FUNCTION_BLOCK FB_Machine
VAR
	// ==============================错误变量=====================================================
	bError				AT%Q*				: BOOL;								// 如果为TRUE，则设备存在错误			（通过输出传递给模拟程序）
	
	// =============================轴相关变量============================================
	fAxisVelo							: LREAL;								// 轴速度，见cAxisVeloAutomatic和cAxisVeloNotAutomatic
		
	// ============================状态机相关变量==================================
	bStarted			AT%Q*				: BOOL;								// 如果为True，则设备进入运行中状态		（通过输出传递给模拟程序）
	bStopped			AT%Q*				: BOOL;								// 如果为True，则设备进入停止状态		（通过输出传递给模拟程序）
	bReset				AT%Q*				: BOOL;								// 如果为True，则设备进入复位中状态		（通过输出传递给模拟程序）
	bAborted			AT%Q*				: BOOL;								// 如果为True，则设备进入中止状态		（通过输出传递给模拟程序）
	bIdle				AT%Q*				: BOOL;								// 如果为True，则设备进入空闲状态		（通过输出传递给模拟程序）
	bAuto				AT%Q*				: BOOL;								// 如果为True，则设备处于自动模式		（通过输出传递给模拟程序）
	bSemi				AT%Q*				: BOOL;								// 如果为True，则设备处于半自动模式		（通过输出传递给模拟程序）
	bManual				AT%Q*				: BOOL;								// 如果为True，则设备处于手动模式		（通过输出传递给模拟程序）
	bMaintenance		AT%Q*				: BOOL;								// 如果为True，则设备处于维护模式		（通过输出传递给模拟程序）
	bStartButtonOff		AT%Q*				: BOOL;								// 如果为True，复位Start按钮			（通过输出传递给模拟程序）

	// =================================对象=======================================
	fbSeparateModule					: FB_SeparatingModule;					// 输送系统
	fbMetalSorting						: FB_SortingModule;						// 金属分拣系统
	fbPlasticSorting					: FB_SortingModule;						// 塑料分拣系统
	fbButtonStart						: FB_SignalHandling;					// 处理启动按钮的信号处理功能块
	fbButtonStop						: FB_SignalHandling;					// 处理停止按钮的信号处理功能块
	fbButtonReset						: FB_SignalHandling;					// 处理复位按钮的信号处理功能块
	fbButtonAbort						: FB_SignalHandling;					// 处理中止按钮的信号处理功能块
	fbButtonAuto						: FB_SignalHandling;					// 处理自动模式按钮的信号处理功能块
	fbButtonSemi						: FB_SignalHandling;					// 处理半自动模式按钮的信号处理功能块
	fbButtonManual						: FB_SignalHandling;					// 处理手动模式按钮的信号处理功能块
	fbButtonMaintenance					: FB_SignalHandling;					// 处理维护模式按钮的信号处理功能块
	fbButtonPower						: FB_SignalHandling;					// 处理使能按钮的信号处理功能块
	fbButtonComprAir					: FB_SignalHandling;					// 处理压缩气缸空气按钮的信号处理功能块
	fbComprAir							: FB_SignalHandling;					// 处理压缩气缸空气的信号处理功能块		（In为fbButtonComprAir的Out）
	fbPowerSupply						: FB_SignalHandling;					// 处理使能的信号处理功能块				（In为fbButtonPower的Out）
	// =================================状态机==========================================
	fbStateMachineAuto					: PS_PackML_StateMachine_Auto;			// 自动模式下的状态机功能块
	fbStateMachineSemiAuto				: PS_PackML_StateMachine_SemiAuto;		// 半自动模式下的状态机功能块
	fbStateMachineManual				: PS_PackML_StateMachine_Manual;		// 手动模式下的状态机功能块
	fbStateMachineMaintenance			: PS_PackML_StateMachine_Maintenance;	// 维护模式下的状态机功能块
	
	ePMLUnitMode						: E_PMLUnitMode := E_PMLUnitMode.IDLE;	// 当前的设备模式
	ePMLUnitModeRequested				: E_PMLUnitMode;						// 请求的设备模式
	fbUnitModeManager					: PS_UnitModeManager;					// 模式切换功能块
	ePMLState							: E_PMLState := E_PMLState.IDLE;		// 当前的设备状态机
	ePMLStateRequested					: E_PMLState;							// 请求的设备状态机
	
	// ===================================其他=====================================
	bInit								: BOOL;									// 如果为TRUE，则设备运行所必须的参数已经初始化完成
	bAxisEnable							: BOOL;									// 如果为TRUE，则轴已经使能
	bManualAxisEnable					: BOOL;									// 如果为TRUE，则轴允许被手动的按钮控制
	fbTriggerStart						: R_TRIG;								// 检测启动按钮的上升沿
	fbTriggerSeparated					: R_TRIG;								// 检测分割完物料的上升沿
	fbTriggerSelectedM					: R_TRIG;								// 检测金属物料被分拣完的上升沿
	fbTriggerSelectedP					: R_TRIG;								// 检测塑料物料被分拣完的上升沿
	nBoxesOnTheWay						: INT;									// 输送带上正在移动的物料
	aClampTemps							: ARRAY[1..100] OF LREAL;				// 正位气缸的温度数据
	aBarrierTemps						: ARRAY[1..100] OF LREAL;				// 栏杆气缸的温度数据
	aMetalTemps							: ARRAY[1..100] OF LREAL;				// 金属气缸的温度数据
	aPlasticTemps						: ARRAY[1..100] OF LREAL;				// 塑料气缸的温度数据
	bStartingIsSetToTrue				: BOOL;									// 如果为TRUE，则启动方法被以TRUE的形式调用
	bResetIsSetToTrue					: BOOL;									// 如果为TRUE，则复位方法被以TRUE的形式调用
	bHaltIsSetToTrue					: BOOL;									// 如果为TRUE，则停止方法被以TRUE的形式调用

	bResetAxis           AT%I*          : BOOL;									// 单独复位轴的报错

END_VAR
VAR CONSTANT
	// ================================轴速度=========================================
	cAxisVeloAutomatic					: LREAL	:= 200.0;						// 自动/半自动模式下轴的运行速度
	cAxisVeloNotAutomatic				: LREAL	:= 100.0;						// 手动/维护模式下轴的运行速度
	
	// ============================= 气缸超时时间参数 =====================================
	cSeparatingTimeOutClamp				: TIME 	:= T#2.5S;						// 正位气缸在位置之间切换判定为超时的时间
	cSeparatingTimeOutBarrier			: TIME 	:= T#3S;						// 栏杆气缸在位置之间切换判定为超时的时间
	cSortingTimeOutCylinder				: TIME 	:= T#3S;						// 分拣气缸在位置之间切换判定为超时的时间
	cSeparatingBarrierAtWork			: TIME 	:= T#3S;						// 栏杆气缸打开的时间
	cSortingMoveAxis					: TIME 	:= T#1S;						// 分拣系统出料皮带运转的时间
	cSortingSensorDelay					: TIME 	:= T#1.4S;						// 对应物料种类传感器检测到之后，到分拣系统气缸推出的延迟时间
END_VAR

// =========================================================
// 关联报错
	
	bError := fbSeparateModule.bAxisError OR fbSeparateModule.bClampError OR fbSeparateModule.bBarrierError
			OR fbMetalSorting.bAxisError OR fbMetalSorting.bCylError 
			OR fbPlasticSorting.bAxisError OR fbPlasticSorting.bCylError;
	
// =========================================================
// 根据不同的模式选择对应轴的速度

	IF (ePMLUnitMode = E_PMLUnitMode.AUTOMATIC) OR (ePMLUnitMode = E_PMLUnitMode.SEMIAUTOMATIC) THEN
		fAxisVelo := cAxisVeloAutomatic;
	ELSE
		fAxisVelo := cAxisVeloNotAutomatic;
	END_IF

// =========================================================
// 检测子系统当中的标志位信号
	
	fbTriggerSeparated(CLK := fbSeparateModule.bSeparated);			// 分割物料完成
	fbTriggerSelectedM(CLK := fbMetalSorting.bSelected);			// 金属物料分拣完成
	fbTriggerSelectedP(CLK := fbPlasticSorting.bSelected);			// 塑料物料分拣完成
						
// =========================================================
// 关联温度
	
	aBarrierTemps 	:= fbSeparateModule.aBarrierTemps;				
	aClampTemps 	:= fbSeparateModule.aClampTemps;
	aMetalTemps 	:= fbMetalSorting.aTemps;
	aPlasticTemps 	:= fbPlasticSorting.aTemps;

// =========================================================
// 方法调用

	// 初始化
	General_Init();

	// 设备请求
	General_Requests();
	
	// 使能、气缸压缩、信号处理功能块的启用
	General_Enable();
	
	// 关联输入
	General_ModuleInputs();
	
	// 关联输出
	General_SetOutput();
	
	// 状态机处理
	General_StateMachine();
	
	// 内部检查
	CylicCheckInternal();
	
	// 复位轴报错（MC_Reset）
	fbSeparateModule.R_Axis.Reset(bResetAxis);
    fbMetalSorting  .R_Axis.Reset(bResetAxis);
	fbPlasticSorting.R_Axis.Reset(bResetAxis);

METHOD PRIVATE CylicCheckInternal
VAR_INPUT
END_VAR


fbSeparateModule.CylicCheck();		// 输送系统内部检查


fbMetalSorting.CylicCheck();		// 金属分拣系统内部检查


fbPlasticSorting.CylicCheck();		// 塑料分拣系统内部检查
END_METHOD

METHOD PRIVATE General_Enable
VAR_INPUT
END_VAR
// =========================================================
// 使能处理

	fbButtonPower.Enable(bEnable := TRUE);			// 启用使能按钮
	fbPowerSupply.Enable(bEnable := TRUE);			// 启用使能按钮输出的信号
	
	fbPowerSupply.bInput := fbButtonPower.bOut;		// 将使能按钮信号的输出传递给使能信号功能块的输入

// =========================================================
// 轴控使能、手动的标志位处理
	
	// 如果设备进入中止状态，则轴使能自动解除							
	IF (ePMLState = E_PMLState.ABORTED) THEN
		bAxisEnable := FALSE;
		
	// 如果使能信号功能块的输出为TRUE，则bAxisEnable为TRUE
	ELSIF fbPowerSupply.bOut THEN
		bAxisEnable := TRUE;
	END_IF
	
	// 允许轴的手动控制：条件：使能上且设备处于运行状态和手动/自动模式
	bManualAxisEnable := fbPowerSupply.bOut AND (ePMLState = E_PMLState.EXECUTE)
						AND ((ePMLUnitMode = E_PMLUnitMode.MANUAL) OR (ePMLUnitMode = E_PMLUnitMode.MAINTENANCE));
						
// =========================================================
// 气缸压缩处理
	
	// 如果不是维护模式，那使能信号的输出传递给气缸加压信号功能块的输入（随着使能信号的输出自动加压）
	IF (ePMLUnitMode <> E_PMLUnitMode.MAINTENANCE) THEN
		fbComprAir.bInput := fbPowerSupply.bOut;
		
	//	气缸加压按钮信号功能块的输出传递给气缸加压信号功能块的输入
	ELSE
		fbComprAir.bInput := fbButtonComprAir.bOut;
	END_IF
	
	// 保持气缸加压信号功能块启用
	fbComprAir.Enable(bEnable := TRUE);
	
	// 维护模式下启用气缸加压按钮信号功能块
	fbButtonComprAir.Enable(bEnable := (ePMLUnitMode = E_PMLUnitMode.MAINTENANCE));

// =========================================================
// 输送系统使能方法的调用

	fbSeparateModule.Enable(bComprAirEnabled	:= fbComprAir.bOut,
							bAxisEnable			:= bAxisEnable,
							bSensorEnable		:= TRUE,
							bManualAxisEnable	:= bManualAxisEnable);

// =========================================================
// 金属分拣系统使能方法的调用

	fbMetalSorting.Enable(	bComprAirEnabled	:= fbComprAir.bOut,
							bAxisEnable			:= bAxisEnable,
							bSensorEnable		:= TRUE,
							bManualAxisEnable	:= bManualAxisEnable);

// =========================================================
// 塑料分拣系统使能方法的调用

	fbPlasticSorting.Enable(bComprAirEnabled	:= fbComprAir.bOut,
							bAxisEnable			:= bAxisEnable,
							bSensorEnable		:= TRUE,
							bManualAxisEnable	:= bManualAxisEnable);

// =========================================================
// 其他信号处理功能块的启用
		
	// 启动按钮：（设备非空闲状态且设备无错误）
	fbButtonStart.Enable(bEnable		:= NOT ((ePMLState = E_PMLState.IDLE) AND bError));
	
	// 停止按钮：（设备运行以及空闲状态下都可以进行停止）
	fbButtonStop.Enable(bEnable 		:= (ePMLState = E_PMLState.EXECUTE) OR (ePMLState = E_PMLState.IDLE));
	
	// 复位按钮：（设备在停止状态下才会被启用）
	fbButtonReset.Enable(bEnable		:= (ePMLState = E_PMLState.STOPPED));
	
	// 使能信号功能块的输出取反传递给中止信号功能块的输入（中止即代表设备掉使能）
	fbButtonAbort.bInput 				:= NOT fbPowerSupply.bOut;
	
	// 中止按钮：（设备在执行、停止中或者复位中才会被启用）
	fbButtonAbort.Enable(bEnable 		:= (ePMLState = E_PMLState.EXECUTE) OR (ePMLState = E_PMLState.STOPPING) OR (ePMLState = E_PMLState.RESETTING));
								
	// 自动模式按钮：（设备在空闲状态下且当前模式非自动模式）
	fbButtonAuto.Enable(bEnable 		:= (ePMLState = E_PMLState.IDLE) AND (ePMLUnitMode <> E_PMLUnitMode.AUTOMATIC));
	
	// 半自动模式按钮：（设备在空闲状态下且当前模式非半自动模式）
	fbButtonSemi.Enable(bEnable 		:= (ePMLState = E_PMLState.IDLE) AND (ePMLUnitMode <> E_PMLUnitMode.SEMIAUTOMATIC));
	
	// 手动模式按钮：（设备在空闲状态下且当前模式非手动模式）
	fbButtonManual.Enable(bEnable 		:= (ePMLState = E_PMLState.IDLE) AND (ePMLUnitMode <> E_PMLUnitMode.MANUAL));
	
	// 维护模式按钮：（设备在空闲状态下且当前模式非维护模式）
	fbButtonMaintenance.Enable(bEnable	:= (ePMLState = E_PMLState.IDLE) AND (ePMLUnitMode <> E_PMLUnitMode.MAINTENANCE));

// =========================================================
END_METHOD

METHOD PRIVATE General_Init
VAR_INPUT
END_VAR
// =========================================================

IF NOT bInit THEN
	
	// 各个子系统的执行必要参数，这些参数都是固定参数，所以只需要传递一次即可
		
		// 传递输送系统正位气缸的超时时间
		fbSeparateModule.tTimeOutOfClamp 			:= cSeparatingTimeOutClamp;
		
		// 传递输送系统栏杆气缸的超时时间
		fbSeparateModule.tTimeOutOfBarrier 			:= cSeparatingTimeOutBarrier;
		
		// 传递输送系统栏杆气缸维持在目标位（打开）的时间
		fbSeparateModule.tBarrierAtWorkPos			:= cSeparatingBarrierAtWork;

		// 传递金属分拣系统正位气缸的超时时间
		fbMetalSorting.tTimeOutOfCylinder 			:= cSortingTimeOutCylinder;		
		
		// 传递金属分拣系统出料皮带运转的时间
		fbMetalSorting.tAxisMovement 				:= cSortingMoveAxis;
		
		// 传递金属物料传感器检测到之后，到金属分拣系统气缸推出的延迟时间
		fbMetalSorting.tDelayOfSensor 				:= cSortingSensorDelay;
		
		// 传递塑料分拣系统正位气缸的超时时间
		fbPlasticSorting.tTimeOutOfCylinder 		:= cSortingTimeOutCylinder;
		
		// 传递塑料分拣系统出料皮带运转的时间
		fbPlasticSorting.tAxisMovement 				:= cSortingMoveAxis;
		
		// 传递塑料物料传感器检测到之后，到塑料分拣系统气缸推出的延迟时间
		fbPlasticSorting.tDelayOfSensor 			:= cSortingSensorDelay;

	// 初始化只执行一次
		bInit := TRUE;
END_IF

// =========================================================
END_METHOD

METHOD PRIVATE General_ModuleInputs
VAR_INPUT
END_VAR
// =========================================================
// 输送系统

	// 如果设备状态为运行状态，则输送系统的bExecute被置为TRUE
	fbSeparateModule.bExecute 			:= (ePMLState = E_PMLState.EXECUTE);
	
	// 每按下一次bStart按钮，输送系统的bSemiStart被置为TRUE，从而保证在半自动模式下，每按下一次bStart启动一次分拣周期
	fbSeparateModule.bSemiStart 		:= fbTriggerStart.Q;
	
	// 传递设定速度到输送系统（运输皮带）当中
	fbSeparateModule.fAxisVelocity 	:= fAxisVelo;

	// 传递皮带上物料的数量到输送系统当中
	fbSeparateModule.nBoxesOnTheWay 	:= nBoxesOnTheWay;
	
	// 通过两个分拣系统物料检测传感器延迟的输出从而判断物料已经到达对应的推出气缸正下方（用于暂停输送皮带的运转）
	fbSeparateModule.P_BoxUndertheCylinderPosition	:= fbPlasticSorting.fbSensorDelay.bOut 		 OR fbMetalSorting .fbSensorDelay.bOut;
	
	// 通过两个分拣系统推出气缸的到达目标位置标志位从而判断对应物料的推出气缸已经工作完成（用于重新启用输送皮带）
	fbSeparateModule.P_CylinderWorkDone				:= fbPlasticSorting.bState_CylinderAtWorkPos OR fbMetalSorting.bState_CylinderAtWorkPos;

// =========================================================
// 金属分拣系统
	
	// 传递设定速度到金属分拣系统（金属出料皮带）当中
	fbMetalSorting.fAxisVelocity 	:= fAxisVelo;

// =========================================================
// 塑料分拣系统

	// 传递设定速度到塑料分拣系统（塑料出料皮带）当中
	fbPlasticSorting.fAxisVelocity 	:= fAxisVelo;
	
// =========================================================
END_METHOD

METHOD PRIVATE General_Requests
VAR_INPUT
END_VAR
// ============================模式=============================

	// 检测启动按钮上升沿
	fbTriggerStart( CLK := fbButtonStart.bOut);
	
	// 如果关闭启动按钮为TRUE，且外部没用按下启动按钮，那么关闭启动按钮自动回归FALSE
	IF bStartButtonOff AND NOT fbButtonStart.bInput THEN
		bStartButtonOff := FALSE;
	END_IF
	
	// 如果检测到启动按钮的上升沿，那么将关闭启动按钮置为TRUE，也只有启动置回，才能将对应的状态传递给ePMLStateRequested
	IF fbTriggerStart.Q THEN
		bStartButtonOff := TRUE;
		
		// 如果设备被中止了，那么状态的请求则为需要清除中
		IF ePMLState = E_PMLState.ABORTED THEN
			ePMLStateRequested := E_PMLState.CLEARING;
		
		// 如果设备停止了，那么状态的请求则为需要复位中	
		ELSIF ePMLState = E_PMLState.STOPPED THEN
			ePMLStateRequested := E_PMLState.RESETTING;
		
		// 如果设备的状态为空闲，且设备已经使能上，那么状态的请求则为需要启动中	
		ELSIF ePMLState = E_PMLState.IDLE AND fbPowerSupply.bOut THEN
			ePMLStateRequested := E_PMLState.STARTING;
		END_IF
		
	// 即使设备没有接收到启动的指令，如果停止按钮按下，那么状态的请求则为需要停止中	
	ELSIF fbButtonStop.bOut THEN
		ePMLStateRequested := E_PMLState.STOPPING;
	
	// 	即使设备没有接收到启动的指令，如果复位按钮按下，那么状态的请求则为需要复位中	
	ELSIF fbButtonReset.bOut THEN
		ePMLStateRequested := E_PMLState.RESETTING;
	END_IF

// ============================状态=============================

	// 如果手动模式按钮按下，那么模式的请求则为手动模式	
	IF fbButtonManual.bOut THEN
		ePMLUnitModeRequested := E_PMLUnitMode.MANUAL;
	
	// 如果自动模式按钮按下，那么模式的请求则为自动模式		
	ELSIF fbButtonAuto.bOut THEN
		ePMLUnitModeRequested := E_PMLUnitMode.AUTOMATIC;
	
	// 如果半自动模式按钮按下，那么模式的请求则为半自动模式		
	ELSIF fbButtonSemi.bOut THEN
		ePMLUnitModeRequested := E_PMLUnitMode.SEMIAUTOMATIC;
	
	// 如果维护模式按钮按下，那么模式的请求则为维护模式		
	ELSIF fbButtonMaintenance.bOut THEN
		ePMLUnitModeRequested := E_PMLUnitMode.MAINTENANCE;
	END_IF
	
	// 如果有任何一个模式按钮的输出模拟，那么会调用模式切换功能块进行模式的切换
	IF fbButtonManual.bOut OR fbButtonAuto.bOut OR fbButtonSemi.bOut OR fbButtonMaintenance.bOut THEN
		fbUnitModeManager(	Execute 		:= TRUE,
							eModeCommand 	:= ePMLUnitModeRequested,
							ePMLState 		:= ePMLState);
	END_IF
	
	// 完成模式切换之后，从模式切换功能块当中传递输出到本地，并将模式切换功能块的Execute置回FALSE
	IF fbUnitModeManager.Done THEN
		ePMLUnitMode := fbUnitModeManager.eModeStatus;
		
		fbUnitModeManager(Execute := FALSE);
	END_IF
	
// =========================================================
END_METHOD

METHOD PRIVATE General_SetOutput
VAR_INPUT
END_VAR
// =========================================================
// 根据PackML状态的枚举体值输出对应的状态标志位

	bStopped 		:= (ePMLState = E_PMLState.STOPPED);
	bStarted 		:= (ePMLState = E_PMLState.EXECUTE);
	bReset 			:= (ePMLState = E_PMLState.RESETTING);
	bAborted 		:= (ePMLState = E_PMLState.ABORTED);
	bIdle 			:= (ePMLState = E_PMLState.IDLE AND fbPowerSupply.bOut);

// =========================================================
// 根据PackML模式的枚举体值输出对应的模式标志位

	bAuto 			:= (ePMLUnitMode = E_PMLUnitMode.AUTOMATIC);
	bSemi 			:= (ePMLUnitMode = E_PMLUnitMode.SEMIAUTOMATIC);
	bManual 		:= (ePMLUnitMode = E_PMLUnitMode.MANUAL);
	bMaintenance 	:= (ePMLUnitMode = E_PMLUnitMode.MAINTENANCE);

// =========================================================
// 输出使能以及压缩气缸信号处理功能块
		
	fbPowerSupply.SetOutput();
	fbComprAir.SetOutput();		

// =========================================================
// 调用各个子系统的输入输出关联方法

	fbSeparateModule.InputOutput();
	fbMetalSorting.InputOutput();
	fbPlasticSorting.InputOutput();

// =========================================================
// 输出各个按钮信号功能块

	fbButtonPower.SetOutput();
	fbButtonComprAir.SetOutput();	
	fbButtonStart.SetOutput();
	fbButtonStop.SetOutput();
	fbButtonReset.SetOutput();
	fbButtonAbort.SetOutput();
	fbButtonAuto.SetOutput();
	fbButtonSemi.SetOutput();
	fbButtonManual.SetOutput();
	fbButtonMaintenance.SetOutput();	
	
// =========================================================
END_METHOD

METHOD PRIVATE General_StateMachine
VAR_INPUT
END_VAR
// =========================================================
	// 模式处理
	
CASE ePMLUnitMode OF
	
	// =========================================================	
	E_PMLUnitMode.AUTOMATIC:		
										  // ePMLStateRequested为 STARTING（在按下启动按钮的时）
				fbStateMachineAuto(	      Start 	:= ePMLStateRequested = E_PMLState.STARTING,	
					
										  // 按下停止按钮时						
									      Stop 	    := fbButtonStop.bOut,	
									
										  // 按下复位按钮时，或者ePMLStateRequested为 RESETTING（停止状态下再次按下启动也可触发）			
									      Reset 	:= fbButtonReset.bOut OR ePMLStateRequested = E_PMLState.RESETTING,		
										  
										  // ePMLStateRequested为 CLEARING（中止状态下按下启动按钮时）
									      Clear 	:= ePMLStateRequested = E_PMLState.CLEARING,				

										  // 按下中止按钮时，或设备在运行的时候出现错误			
									      Abort   	:= fbButtonAbort.bOut OR (bError AND ePMLState = E_PMLState.EXECUTE),	
										  
                                          ePMLState => ePMLState );

				
				Operating_Automatic();

	// =========================================================	
	E_PMLUnitMode.MANUAL:	
	
				// 同上
				fbStateMachineManual(     Start 	:= ePMLStateRequested = E_PMLState.STARTING,
										  Stop 	    := fbButtonStop.bOut,
										  Reset 	:= fbButtonReset.bOut OR ePMLStateRequested = E_PMLState.RESETTING,
										  Clear 	:= ePMLStateRequested = E_PMLState.CLEARING,
										  Abort 	:= fbButtonAbort.bOut OR (bError AND ePMLState = E_PMLState.EXECUTE),
                                          ePMLState => ePMLState);

				
				Operating_Manual();
	
	// =========================================================						
	E_PMLUnitMode.SEMIAUTOMATIC:	

				// 同上
				fbStateMachineSemiAuto(	  Start 	:= ePMLStateRequested = E_PMLState.STARTING,
									 	  Stop 	    := fbButtonStop.bOut,
										  Reset 	:= fbButtonReset.bOut OR ePMLStateRequested = E_PMLState.RESETTING,
										  Clear 	:= ePMLStateRequested = E_PMLState.CLEARING,
										  Abort 	:= fbButtonAbort.bOut OR (bError AND ePMLState = E_PMLState.EXECUTE),
                                          ePMLState => ePMLState);

				
				Operating_Semiautomatic();
	
	// =========================================================						
	E_PMLUnitMode.MAINTENANCE:	

				// 同上
				fbStateMachineMaintenance(Start 	:= ePMLStateRequested = E_PMLState.STARTING,
										  Stop      := fbButtonStop.bOut,
										  Reset 	:= fbButtonReset.bOut OR ePMLStateRequested = E_PMLState.RESETTING,
										  Clear 	:= ePMLStateRequested = E_PMLState.CLEARING,
										  Abort 	:= fbButtonAbort.bOut OR (bError AND ePMLState = E_PMLState.EXECUTE),
                                          ePMLState => ePMLState);

				
				Operating_Maintenance();
END_CASE

// =========================================================
END_METHOD

METHOD PRIVATE Operating_Automatic
VAR_INPUT
END_VAR
// =========================================================

CASE ePMLState OF
	
	// ========================空闲状态=================================
	E_PMLState.IDLE:
	
				// 如果上一个周期中，是用复位来进入空闲状态时，那么先让各个子系统的复位方法以FALSE的形式调用。顺便将StateComplete置回FALSE
				IF bResetIsSetToTrue THEN
					bResetIsSetToTrue := FALSE;
					
					fbSeparateModule.Reset(bReset := FALSE);							
					fbMetalSorting.Reset(bReset := FALSE);
					fbPlasticSorting.Reset(bReset := FALSE);
					
					fbStateMachineAuto.StateComplete := FALSE;	
				END_IF
	
	// ========================启动中状态================================
	E_PMLState.STARTING:
	
				// 以TRUE的形式调用各个子系统的Starting方法
				IF NOT bStartingIsSetToTrue THEN
					bStartingIsSetToTrue := TRUE;
					
					fbSeparateModule.Starting(bStarting := TRUE);
					fbMetalSorting.Starting(bStarting := TRUE);
					fbPlasticSorting.Starting(bStarting := TRUE);
				END_IF
				
				// 如果各个子系统未完成启动的流程，则继续以TRUE的形式调用各个子系统的Starting方法
				IF NOT fbSeparateModule.bState_StartingDone THEN		
					fbSeparateModule.Starting(bStarting := TRUE);
				END_IF	
				IF NOT fbMetalSorting.bState_StartingDone THEN
					fbMetalSorting.Starting(bStarting := TRUE);
				END_IF				
				IF NOT fbPlasticSorting.bState_StartingDone THEN
					fbPlasticSorting.Starting(bStarting := TRUE);
				END_IF

				// 如果所有子系统都完成了启动，那StateComplete则为TRUE。代表启动完成。状态会经过状态机功能块自动进入EXECUTE
				IF fbSeparateModule.bState_StartingDone AND fbMetalSorting.bState_StartingDone AND fbPlasticSorting.bState_StartingDone THEN
					fbStateMachineAuto.StateComplete := TRUE;
				END_IF

	// ==========================执行中状态===============================
	E_PMLState.EXECUTE:	
				
				// 进入运行状态之后，先将bStartingIsSetToTrue置为FALSE，再将各个子系统的启动方法以FALSE调用，同时StateComplete置为FALSE
				IF bStartingIsSetToTrue THEN
					bStartingIsSetToTrue := FALSE;
					
					fbSeparateModule.Starting(bStarting := FALSE);
					fbMetalSorting.Starting(bStarting := FALSE);	
					fbPlasticSorting.Starting(bStarting := FALSE);
					
					fbStateMachineAuto.StateComplete := FALSE;
				END_IF
				
				// 调用各个子系统的自动方法
				fbSeparateModule.Automatic();
				fbMetalSorting.Automatic();
				fbPlasticSorting.Automatic();
				
				// 如果检测到被分割物料的上升沿，那么nBoxesOnTheWay会加1，代表输送带上有一个物料正在运输
				IF fbTriggerSeparated.Q THEN
					nBoxesOnTheWay := nBoxesOnTheWay + 1;
				END_IF
				
				// 如果检测到金属物料被分拣完成的上升沿，那么nBoxesOnTheWay会减1，代表输送带上少了一个正在运输的物料
				IF fbTriggerSelectedM.Q THEN
					nBoxesOnTheWay := nBoxesOnTheWay - 1;
				END_IF
				
				// 如果检测到塑料物料被分拣完成的上升沿，那么nBoxesOnTheWay会减1，代表输送带上少了一个正在运输的物料
				IF fbTriggerSelectedP.Q THEN
					nBoxesOnTheWay := nBoxesOnTheWay - 1;
				END_IF
						
	// =========================中止中状态================================
	E_PMLState.ABORTING:

				// 进入中止中状态之后，先将bHaltIsSetToTrue置为TRUE，再将各个子系统的Halt方法以TRUE调用
				IF NOT bHaltIsSetToTrue THEN
					bHaltIsSetToTrue := TRUE;
					
					fbSeparateModule.Halt(bHalt := TRUE);
					fbMetalSorting.Halt(bHalt := TRUE);
					fbPlasticSorting.Halt(bHalt := TRUE);
				END_IF

				// 如果各个子系统未完成停止的流程，则继续以TRUE的形式继续调用各个子系统的Halt方法
				IF NOT fbSeparateModule.bState_HaltDone THEN
					fbSeparateModule.Halt(bHalt := TRUE);
				END_IF		
				IF NOT fbMetalSorting.bState_HaltDone THEN
					fbMetalSorting.Halt(bHalt := TRUE);
				END_IF				
				IF NOT fbPlasticSorting.bState_HaltDone THEN
					fbPlasticSorting.Halt(bHalt := TRUE);
				END_IF

				// 如果所有子系统都停止了，那StateComplete则为TRUE。代表中止完成。状态会经过状态机功能块自动进入ABORTED
				IF fbSeparateModule.bState_HaltDone AND fbMetalSorting.bState_HaltDone AND fbPlasticSorting.bState_HaltDone THEN
					fbStateMachineAuto.StateComplete := TRUE;
				END_IF
	
	// ========================中止状态=================================
	E_PMLState.ABORTED:
				
				// 进入中止状态之后，先将bHaltIsSetToTrue置回FALSE，再将各个子系统的Halt方法以FALSE调用
				IF bHaltIsSetToTrue THEN
					bHaltIsSetToTrue := FALSE;
					
					fbSeparateModule.Halt(bHalt := FALSE);
					fbMetalSorting.Halt(bHalt := FALSE);
					fbPlasticSorting.Halt(bHalt := FALSE);
				END_IF
				
				// 将StateComplete置回FALSE
				IF fbStateMachineAuto.StateComplete THEN
					fbStateMachineAuto.StateComplete := FALSE;
				END_IF
	
	// =======================清除中状态================================
	E_PMLState.CLEARING:
				
				// 将StateComplete置为TRUE，这里清除中的过程是用Reseting代替
				fbStateMachineAuto.StateComplete := TRUE;
	
	// =========================正常的停止中状态================================
	E_PMLState.STOPPING:	
				
				// 如果检测到被分割物料的上升沿，那么nBoxesOnTheWay会加1，代表输送带上有一个物料正在运输
				IF fbTriggerSeparated.Q THEN
					nBoxesOnTheWay := nBoxesOnTheWay + 1;
				END_IF		
		
				// 如果检测到金属物料被分拣完成的上升沿，那么nBoxesOnTheWay会减1，代表输送带上少了一个正在运输的物料
				IF fbTriggerSelectedM.Q THEN
					nBoxesOnTheWay := nBoxesOnTheWay - 1;
				END_IF
				
				// 如果检测到塑料物料被分拣完成的上升沿，那么nBoxesOnTheWay会减1，代表输送带上少了一个正在运输的物料
				IF fbTriggerSelectedP.Q THEN
					nBoxesOnTheWay := nBoxesOnTheWay - 1;
				END_IF
				
					// 只有当nBoxesOnTheWay为0且bHaltIsSetToTrue为FALSE（没用以TRUE调用过Halt方法）的时候，将bHaltIsSetToTrue置为TRUE
				IF (nBoxesOnTheWay = 0) AND NOT bHaltIsSetToTrue THEN
					bHaltIsSetToTrue := TRUE;
				END_IF
				
				// 如果输送系统没用完成停止，或者输送带上仍然有物料，那么继续调用输送系统的自动方法等待该流程执行完毕。当nBoxesOnTheWay为0，以TRUE调用输送系统的Halt方法
				IF NOT fbSeparateModule.bState_HaltDone OR (nBoxesOnTheWay <> 0) THEN
					fbSeparateModule.Automatic();
					
					IF (nBoxesOnTheWay = 0) THEN
						fbSeparateModule.Halt(bHalt := TRUE);
					END_IF
				END_IF
				
				// 如果输送系统没用完成停止，或者输送带上仍然有物料，那么继续调用输送系统的自动方法等待该流程执行完毕。当nBoxesOnTheWay为0，以TRUE调用金属分拣系统的Halt方法
				IF NOT fbMetalSorting.bState_HaltDone OR (nBoxesOnTheWay <> 0) THEN
					fbMetalSorting.Automatic();
					
					IF (nBoxesOnTheWay = 0) THEN
						fbMetalSorting.Halt(bHalt := TRUE);
					END_IF
				END_IF
				
				// 如果输送系统没用完成停止，或者输送带上仍然有物料，那么继续调用输送系统的自动方法等待该流程执行完毕。当nBoxesOnTheWay为0，以TRUE调用塑料分拣系统的Halt方法
				IF NOT fbPlasticSorting.bState_HaltDone OR (nBoxesOnTheWay <> 0) THEN
					fbPlasticSorting.Automatic();
					
					IF (nBoxesOnTheWay = 0) THEN
						fbPlasticSorting.Halt(bHalt := TRUE);
					END_IF
				END_IF
				
				// 如果各个子系统都完成停止了，且输送带上没有物料了，StateComplete才会被置为TRUE，代表停止完成。状态会经过状态机功能块自动进入STOPPED
				IF fbSeparateModule.bState_HaltDone AND fbMetalSorting.bState_HaltDone
				AND fbPlasticSorting.bState_HaltDone AND (nBoxesOnTheWay = 0) THEN
					fbStateMachineAuto.StateComplete := TRUE;
				END_IF
					
	// ===========================停止状态==============================
	E_PMLState.STOPPED:	

				// 进入停止状态之后，先将bHaltIsSetToTrue置回FALSE，再将各个子系统的Halt方法以FALSE调用
				IF bHaltIsSetToTrue THEN
					bHaltIsSetToTrue := FALSE;
					
					fbSeparateModule.Halt(bHalt := FALSE);	
					fbMetalSorting.Halt(bHalt := FALSE);			
					fbPlasticSorting.Halt(bHalt := FALSE);
				END_IF

				// 将StateComplete置回FALSE
				IF fbStateMachineAuto.StateComplete THEN
					fbStateMachineAuto.StateComplete := FALSE;	
				END_IF

	// =========================复位中状态================================
	E_PMLState.RESETTING:	

				// 进入复位中状态之后，先将bResetIsSetToTrue置为TRUE，再将各个子系统的Reset方法以TRUE调用
				IF NOT bResetIsSetToTrue THEN
					bResetIsSetToTrue := TRUE;
					
					fbSeparateModule.Reset(bReset := TRUE);							
					fbMetalSorting.Reset(bReset := TRUE);
					fbPlasticSorting.Reset(bReset := TRUE);
				END_IF
				
				// 如果各个子系统未完成复位的流程，则继续以TRUE的形式继续调用各个子系统的Reset方法
				IF NOT fbSeparateModule.bState_ResetDone THEN
					fbSeparateModule.Reset(bReset := TRUE);
				END_IF			
				IF NOT fbMetalSorting.bState_ResetDone THEN
					fbMetalSorting.Reset(bReset := TRUE);
				END_IF				
				IF NOT fbPlasticSorting.bState_ResetDone THEN
					fbPlasticSorting.Reset(bReset := TRUE);
				END_IF
				
				// 如果各个子系统都完成复位了，且所有气缸都回到基始位了，那么nBoxesOnTheWay也一并清零。同时，将StateComplete置为TRUE
				IF fbSeparateModule.bState_ResetDone AND fbMetalSorting.bState_ResetDone AND fbPlasticSorting.bState_ResetDone 
				AND fbSeparateModule.bState_ClampAtBasePos AND fbSeparateModule.bState_BarrierAtBasePos
				AND fbMetalSorting.bState_CylinderAtBasePos AND fbPlasticSorting.bState_CylinderAtBasePos THEN
					nBoxesOnTheWay 						:= 0;
					fbStateMachineAuto.StateComplete 	:= TRUE;
				END_IF
END_CASE

// =========================================================
END_METHOD

METHOD PRIVATE Operating_Maintenance
VAR_INPUT
END_VAR
// =========================================================

CASE ePMLState OF
	
	// ========================空闲状态=================================
	E_PMLState.IDLE:		

				// 如果上一个周期中，是用复位来进入空闲状态时，那么先让各个子系统的复位方法以FALSE的形式调用。顺便将StateComplete置回FALSE
				IF bResetIsSetToTrue THEN
					bResetIsSetToTrue := FALSE;
					
					fbSeparateModule.Reset(bReset := FALSE);
					fbMetalSorting.Reset(bReset := FALSE);
					fbPlasticSorting.Reset(bReset := FALSE);
					
					fbStateMachineMaintenance.StateComplete := FALSE;
				END_IF
	
	// ========================启动中状态================================
	E_PMLState.STARTING:	

				// 以TRUE的形式调用各个子系统的Starting方法
				IF NOT bStartingIsSetToTrue THEN
					bStartingIsSetToTrue := TRUE;
					
					fbSeparateModule.Starting(bStarting := TRUE);
					fbMetalSorting.Starting(bStarting := TRUE);
					fbPlasticSorting.Starting(bStarting := TRUE);
				END_IF
				
				// 如果各个子系统未完成启动的流程，则继续以TRUE的形式调用各个子系统的Starting方法
				IF NOT fbSeparateModule.bState_StartingDone THEN
					fbSeparateModule.Starting(bStarting := TRUE);
				END_IF			
				IF NOT fbMetalSorting.bState_StartingDone THEN
					fbMetalSorting.Starting(bStarting := TRUE);
				END_IF				
				IF NOT fbPlasticSorting.bState_StartingDone THEN
					fbPlasticSorting.Starting(bStarting := TRUE);
				END_IF

				// 如果所有子系统都完成了启动，那StateComplete则为TRUE。代表启动完成。状态会经过状态机功能块自动进入EXECUTE
				IF fbSeparateModule.bState_StartingDone AND fbMetalSorting.bState_StartingDone AND fbPlasticSorting.bState_StartingDone THEN
					fbStateMachineMaintenance.StateComplete := TRUE;
				END_IF

	// ==========================执行中状态===============================
	E_PMLState.EXECUTE:	

				// 进入运行状态之后，先将bStartingIsSetToTrue置为FALSE，再将各个子系统的启动方法以FALSE调用，同时StateComplete置为FALSE
				IF bStartingIsSetToTrue THEN
					bStartingIsSetToTrue := FALSE;
					
					fbSeparateModule.Starting(bStarting := FALSE);
					fbMetalSorting.Starting(bStarting := FALSE);	
					fbPlasticSorting.Starting(bStarting := FALSE);
					
					fbStateMachineMaintenance.StateComplete := FALSE;
				END_IF
				
				// 调用各个子系统的维护方法
				fbSeparateModule.Maintenance();
				fbMetalSorting.Maintenance();
				fbPlasticSorting.Maintenance();
						
	// =========================中止中状态================================
	E_PMLState.ABORTING:	

				// 进入中止中状态之后，先将bHaltIsSetToTrue置为TRUE，再将各个子系统的Halt方法以TRUE调用
				IF NOT bHaltIsSetToTrue THEN
					bHaltIsSetToTrue := TRUE;
					
					fbSeparateModule.Halt(bHalt := TRUE);
					fbMetalSorting.Halt(bHalt := TRUE);
					fbPlasticSorting.Halt(bHalt := TRUE);
				END_IF

				// 如果各个子系统未完成停止的流程，则继续以TRUE的形式继续调用各个子系统的Halt方法
				IF NOT fbSeparateModule.bState_HaltDone THEN
					fbSeparateModule.Halt(bHalt := TRUE);
				END_IF				
				IF NOT fbMetalSorting.bState_HaltDone THEN
					fbMetalSorting.Halt(bHalt := TRUE);
				END_IF				
				IF NOT fbPlasticSorting.bState_HaltDone THEN
					fbPlasticSorting.Halt(bHalt := TRUE);
				END_IF

				// 如果所有子系统都停止了，那StateComplete则为TRUE。代表中止完成。状态会经过状态机功能块自动进入ABORTED
				IF fbSeparateModule.bState_HaltDone AND fbMetalSorting.bState_HaltDone AND fbPlasticSorting.bState_HaltDone THEN
					fbStateMachineMaintenance.StateComplete := TRUE;
				END_IF
	
	// ========================中止状态=================================
	E_PMLState.ABORTED:	

				// 进入中止状态之后，先将bHaltIsSetToTrue置回FALSE，再将各个子系统的Halt方法以FALSE调用
				IF bHaltIsSetToTrue THEN
					bHaltIsSetToTrue := FALSE;
					
					fbSeparateModule.Halt(bHalt := FALSE);
					fbMetalSorting.Halt(bHalt := FALSE);
					fbPlasticSorting.Halt(bHalt := FALSE);
				END_IF

				// 将StateComplete置回FALSE
				IF fbStateMachineMaintenance.StateComplete THEN
					fbStateMachineMaintenance.StateComplete := FALSE;
				END_IF
	
	// =======================清除中状态================================
	E_PMLState.CLEARING:
				
				// 将StateComplete置为TRUE，这里清除中的过程是用Reseting代替
				fbStateMachineAuto.StateComplete := TRUE;
	
	// =========================正常的停止中状态================================
	E_PMLState.STOPPING:	

				// 只有当bHaltIsSetToTrue为FALSE（没用以TRUE调用过Halt方法）的时候，才会以TRUE调用各个子系统的Halt方法
				IF NOT bHaltIsSetToTrue THEN
					bHaltIsSetToTrue := TRUE;

					fbSeparateModule.Halt(bHalt := TRUE);				
					fbMetalSorting.Halt(bHalt := TRUE);				
					fbPlasticSorting.Halt(bHalt := TRUE);				
				END_IF

				// 如果各个子系统没用完成停止了。那么继续以TRUE调用输送系统的Halt方法
				IF NOT fbSeparateModule.bState_HaltDone THEN
					fbSeparateModule.Halt(bHalt := TRUE);
				END_IF				
				IF NOT fbMetalSorting.bState_HaltDone THEN
					fbMetalSorting.Halt(bHalt := TRUE);
				END_IF				
				IF NOT fbPlasticSorting.bState_HaltDone THEN
					fbPlasticSorting.Halt(bHalt := TRUE);
				END_IF

				// 如果各个子系统都完成停止了，StateComplete才会被置为TRUE，代表停止完成。状态会经过状态机功能块自动进入STOPPED
				IF fbSeparateModule.bState_HaltDone AND fbMetalSorting.bState_HaltDone AND fbPlasticSorting.bState_HaltDone THEN
						fbStateMachineMaintenance.StateComplete := TRUE;
				END_IF
					
	// ===========================停止状态==============================
	E_PMLState.STOPPED:	

				// 进入停止状态之后，先将bHaltIsSetToTrue置回FALSE，再将各个子系统的Halt方法以FALSE调用
				IF bHaltIsSetToTrue THEN
					bHaltIsSetToTrue := FALSE;
					
					fbSeparateModule.Halt(bHalt := FALSE);	
					fbMetalSorting.Halt(bHalt := FALSE);			
					fbPlasticSorting.Halt(bHalt := FALSE);
				END_IF

				// 将StateComplete置回FALSE
				IF fbStateMachineMaintenance.StateComplete THEN
					fbStateMachineMaintenance.StateComplete := FALSE;
				END_IF

	// =========================复位中状态================================
	E_PMLState.RESETTING:	

				// 进入复位中状态之后，先将bResetIsSetToTrue置为TRUE，再将各个子系统的Reset方法以TRUE调用
				IF NOT bResetIsSetToTrue THEN
					bResetIsSetToTrue := TRUE;
					
					fbSeparateModule.Reset(bReset := TRUE);							
					fbMetalSorting.Reset(bReset := TRUE);
					fbPlasticSorting.Reset(bReset := TRUE);
				END_IF
				
				// 如果各个子系统未完成复位的流程，则继续以TRUE的形式继续调用各个子系统的Reset方法
				IF NOT fbSeparateModule.bState_ResetDone THEN
					fbSeparateModule.Reset(bReset := TRUE);
				END_IF				
				IF NOT fbMetalSorting.bState_ResetDone THEN
					fbMetalSorting.Reset(bReset := TRUE);
				END_IF				
				IF NOT fbPlasticSorting.bState_ResetDone THEN
					fbPlasticSorting.Reset(bReset := TRUE);
				END_IF
				
				// 如果各个子系统都完成复位了，且所有气缸都回到基始位了，那么将StateComplete置为TRUE
				IF fbSeparateModule.bState_ResetDone AND fbMetalSorting.bState_ResetDone AND fbPlasticSorting.bState_ResetDone 
				AND fbSeparateModule.bState_ClampAtBasePos AND fbSeparateModule.bState_BarrierAtBasePos
				AND fbMetalSorting.bState_CylinderAtBasePos AND fbPlasticSorting.bState_CylinderAtBasePos THEN
					fbStateMachineMaintenance.StateComplete := TRUE;
				END_IF
END_CASE

// =========================================================
END_METHOD

METHOD PRIVATE Operating_Manual
VAR_INPUT
END_VAR
// =========================================================

CASE ePMLState OF
	
	// ========================空闲状态=================================
	E_PMLState.IDLE:		

				// 如果上一个周期中，是用复位来进入空闲状态时，那么先让各个子系统的复位方法以FALSE的形式调用。顺便将StateComplete置回FALSE
				IF bResetIsSetToTrue THEN
					bResetIsSetToTrue := FALSE;
					
					fbSeparateModule.Reset(bReset := FALSE);
					fbMetalSorting.Reset(bReset := FALSE);
					fbPlasticSorting.Reset(bReset := FALSE);
					
					fbStateMachineManual.StateComplete := FALSE;
				END_IF
	
	// ========================启动中状态================================
	E_PMLState.STARTING:	

				// 以TRUE的形式调用各个子系统的Starting方法
				IF NOT bStartingIsSetToTrue THEN
					bStartingIsSetToTrue := TRUE;
					
					fbSeparateModule.Starting(bStarting := TRUE);
					fbMetalSorting.Starting(bStarting := TRUE);
					fbPlasticSorting.Starting(bStarting := TRUE);
				END_IF

				// 如果各个子系统未完成启动的流程，则继续以TRUE的形式调用各个子系统的Starting方法
				IF NOT fbSeparateModule.bState_StartingDone THEN
					fbSeparateModule.Starting(bStarting := TRUE);
				END_IF				
				IF NOT fbMetalSorting.bState_StartingDone THEN
					fbMetalSorting.Starting(bStarting := TRUE);
				END_IF				
				IF NOT fbPlasticSorting.bState_StartingDone THEN
					fbPlasticSorting.Starting(bStarting := TRUE);
				END_IF

				// 如果所有子系统都完成了启动，那StateComplete则为TRUE。代表启动完成。状态会经过状态机功能块自动进入EXECUTE
				IF fbSeparateModule.bState_StartingDone AND fbMetalSorting.bState_StartingDone AND fbPlasticSorting.bState_StartingDone THEN
					fbStateMachineManual.StateComplete := TRUE;
				END_IF

	// ==========================执行中状态===============================
	E_PMLState.EXECUTE:	

				// 进入运行状态之后，先将bStartingIsSetToTrue置为FALSE，再将各个子系统的启动方法以FALSE调用，同时StateComplete置为FALSE
				IF bStartingIsSetToTrue THEN
					bStartingIsSetToTrue := FALSE;
					
					fbSeparateModule.Starting(bStarting := FALSE);
					fbMetalSorting.Starting(bStarting := FALSE);
					fbPlasticSorting.Starting(bStarting := FALSE);
					
					fbStateMachineManual.StateComplete := FALSE;
				END_IF
				
				// 调用各个子系统的手动方法
				fbSeparateModule.Manual();
				fbMetalSorting.Manual();
				fbPlasticSorting.Manual();
						
	// =========================中止中状态================================
	E_PMLState.ABORTING:	

				// 进入中止中状态之后，先将bHaltIsSetToTrue置为TRUE，再将各个子系统的Halt方法以TRUE调用
				IF NOT bHaltIsSetToTrue THEN
					bHaltIsSetToTrue := TRUE;
					
					fbSeparateModule.Halt(bHalt := TRUE);
					fbMetalSorting.Halt(bHalt := TRUE);
					fbPlasticSorting.Halt(bHalt := TRUE);
				END_IF

				// 如果各个子系统未完成停止的流程，则继续以TRUE的形式继续调用各个子系统的Halt方法
				IF NOT fbSeparateModule.bState_HaltDone THEN
					fbSeparateModule.Halt(bHalt := TRUE);
				END_IF				
				IF NOT fbMetalSorting.bState_HaltDone THEN
					fbMetalSorting.Halt(bHalt := TRUE);
				END_IF				
				IF NOT fbPlasticSorting.bState_HaltDone THEN
					fbPlasticSorting.Halt(bHalt := TRUE);
				END_IF

				// 如果所有子系统都停止了，那StateComplete则为TRUE。代表中止完成。状态会经过状态机功能块自动进入ABORTED
				IF fbSeparateModule.bState_HaltDone AND fbMetalSorting.bState_HaltDone AND fbPlasticSorting.bState_HaltDone THEN
					fbStateMachineManual.StateComplete := TRUE;
				END_IF
	
	// ========================中止状态=================================
	E_PMLState.ABORTED:	

				// 进入中止状态之后，先将bHaltIsSetToTrue置回FALSE，再将各个子系统的Halt方法以FALSE调用
				IF bHaltIsSetToTrue THEN
					bHaltIsSetToTrue := FALSE;
					
					fbSeparateModule.Halt(bHalt := FALSE);
					fbMetalSorting.Halt(bHalt := FALSE);
					fbPlasticSorting.Halt(bHalt := FALSE);
				END_IF

				// 将StateComplete置回FALSE
				IF fbStateMachineManual.StateComplete THEN
					fbStateMachineManual.StateComplete := FALSE;
				END_IF
	
	// =======================清除中状态================================
	E_PMLState.CLEARING:
				
				// 将StateComplete置为TRUE，这里清除中的过程是用Reseting代替
				fbStateMachineAuto.StateComplete := TRUE;
	
	// =========================正常的停止中状态================================
	E_PMLState.STOPPING:	

				// 只有当bHaltIsSetToTrue为FALSE（没用以TRUE调用过Halt方法）的时候，才会以TRUE调用各个子系统的Halt方法
				IF NOT bHaltIsSetToTrue THEN
					bHaltIsSetToTrue := TRUE;
					
					fbSeparateModule.Halt(bHalt := TRUE);				
					fbMetalSorting.Halt(bHalt := TRUE);				
					fbPlasticSorting.Halt(bHalt := TRUE);	
				END_IF

				// 如果各个子系统没用完成停止了。那么继续以TRUE调用输送系统的Halt方法
				IF NOT fbSeparateModule.bState_HaltDone THEN
					fbSeparateModule.Halt(bHalt := TRUE);
				END_IF				
				IF NOT fbMetalSorting.bState_HaltDone THEN
					fbMetalSorting.Halt(bHalt := TRUE);
				END_IF			
				IF NOT fbPlasticSorting.bState_HaltDone THEN
					fbPlasticSorting.Halt(bHalt := TRUE);
				END_IF

				// 如果各个子系统都完成停止了，StateComplete才会被置为TRUE，代表停止完成。状态会经过状态机功能块自动进入STOPPED
				IF fbSeparateModule.bState_HaltDone AND fbMetalSorting.bState_HaltDone AND fbPlasticSorting.bState_HaltDone THEN
					fbStateMachineManual.StateComplete := TRUE;
				END_IF
					
	// ===========================停止状态==============================
	E_PMLState.STOPPED:	
	
				// 进入停止状态之后，先将bHaltIsSetToTrue置回FALSE，再将各个子系统的Halt方法以FALSE调用
				IF bHaltIsSetToTrue THEN
					bHaltIsSetToTrue := FALSE;
					
					fbSeparateModule.Halt(bHalt := FALSE);
					fbMetalSorting.Halt(bHalt := FALSE);
					fbPlasticSorting.Halt(bHalt := FALSE);
				END_IF

				// 将StateComplete置回FALSE
				IF fbStateMachineManual.StateComplete THEN
					fbStateMachineManual.StateComplete := FALSE;
				END_IF
				
	// =========================复位中状态================================
	E_PMLState.RESETTING:	

				// 进入复位中状态之后，先将bResetIsSetToTrue置为TRUE，再将各个子系统的Reset方法以TRUE调用
				IF NOT bResetIsSetToTrue THEN
					bResetIsSetToTrue := TRUE;
					
					fbSeparateModule.Reset(bReset := TRUE);							
					fbMetalSorting.Reset(bReset := TRUE);
					fbPlasticSorting.Reset(bReset := TRUE);
				END_IF
				
				// 如果各个子系统未完成复位的流程，则继续以TRUE的形式继续调用各个子系统的Reset方法
				IF NOT fbSeparateModule.bState_ResetDone THEN
					fbSeparateModule.Reset(bReset := TRUE);
				END_IF				
				IF NOT fbMetalSorting.bState_ResetDone THEN
					fbMetalSorting.Reset(bReset := TRUE);
				END_IF				
				IF NOT fbPlasticSorting.bState_ResetDone THEN
					fbPlasticSorting.Reset(bReset := TRUE);
				END_IF

				// 如果各个子系统都完成复位了，且所有气缸都回到基始位了，那么将StateComplete置为TRUE				
				IF fbSeparateModule.bState_ResetDone AND fbMetalSorting.bState_ResetDone AND fbPlasticSorting.bState_ResetDone 
				AND fbSeparateModule.bState_ClampAtBasePos AND fbSeparateModule.bState_BarrierAtBasePos
				AND fbMetalSorting.bState_CylinderAtBasePos AND fbPlasticSorting.bState_CylinderAtBasePos THEN
					fbStateMachineManual.StateComplete := TRUE;
				END_IF
END_CASE

// =========================================================
END_METHOD

METHOD PRIVATE Operating_Semiautomatic
VAR_INPUT
END_VAR
// =========================================================

CASE ePMLState OF
	
	// ========================空闲状态=================================
	E_PMLState.IDLE:		

				// 如果上一个周期中，是用复位来进入空闲状态时，那么先让各个子系统的复位方法以FALSE的形式调用。顺便将StateComplete置回FALSE
				IF bResetIsSetToTrue THEN
					bResetIsSetToTrue := FALSE;
					
					fbSeparateModule.Reset(bReset := FALSE);
					fbMetalSorting.Reset(bReset := FALSE);
					fbPlasticSorting.Reset(bReset := FALSE);
					
					fbStateMachineSemiAuto.StateComplete := FALSE;
				END_IF
	
	// ========================启动中状态================================
	E_PMLState.STARTING:	

				// 以TRUE的形式调用各个子系统的Starting方法
				IF NOT bStartingIsSetToTrue THEN
					bStartingIsSetToTrue := TRUE;
					
					fbSeparateModule.Starting(bStarting := TRUE);
					fbMetalSorting.Starting(bStarting := TRUE);
					fbPlasticSorting.Starting(bStarting := TRUE);
				END_IF

				// 如果各个子系统未完成启动的流程，则继续以TRUE的形式调用各个子系统的Starting方法
				IF NOT fbSeparateModule.bState_StartingDone THEN
					fbSeparateModule.Starting(bStarting := TRUE);
				END_IF			
				IF NOT fbMetalSorting.bState_StartingDone THEN
					fbMetalSorting.Starting(bStarting := TRUE);
				END_IF			
				IF NOT fbPlasticSorting.bState_StartingDone THEN
					fbPlasticSorting.Starting(bStarting := TRUE);
				END_IF

				// 如果所有子系统都完成了启动，那StateComplete则为TRUE。代表启动完成。状态会经过状态机功能块自动进入EXECUTE
				IF fbSeparateModule.bState_StartingDone AND fbMetalSorting.bState_StartingDone AND fbPlasticSorting.bState_StartingDone THEN
					fbStateMachineSemiAuto.StateComplete := TRUE;
				END_IF

	// ==========================执行中状态===============================
	E_PMLState.EXECUTE:	

				// 进入运行状态之后，先将bStartingIsSetToTrue置为FALSE，再将各个子系统的启动方法以FALSE调用，同时StateComplete置为FALSE
				IF bStartingIsSetToTrue THEN
					bStartingIsSetToTrue := FALSE;
					
					fbSeparateModule.Starting(bStarting := FALSE);
					fbMetalSorting.Starting(bStarting := FALSE);
					fbPlasticSorting.Starting(bStarting := FALSE);
					
					fbStateMachineSemiAuto.StateComplete := FALSE;
				END_IF
				
				// 调用各个子系统的半自动方法
				fbSeparateModule.Semiautomatic();
				fbMetalSorting.Semiautomatic();
				fbPlasticSorting.Semiautomatic();
				
				// 如果检测到被分割物料的上升沿，那么nBoxesOnTheWay会加1，代表输送带上有一个物料正在运输
				IF fbTriggerSeparated.Q THEN
					nBoxesOnTheWay := nBoxesOnTheWay + 1;
				END_IF
				
				// 如果检测到金属物料被分拣完成的上升沿，那么nBoxesOnTheWay会减1，代表输送带上少了一个正在运输的物料
				IF fbTriggerSelectedM.Q THEN
					nBoxesOnTheWay := nBoxesOnTheWay - 1;
				END_IF
				
				// 如果检测到塑料物料被分拣完成的上升沿，那么nBoxesOnTheWay会减1，代表输送带上少了一个正在运输的物料
				IF fbTriggerSelectedP.Q THEN
					nBoxesOnTheWay := nBoxesOnTheWay - 1;
				END_IF
						
	// =========================中止中状态================================
	E_PMLState.ABORTING:	

				// 进入中止中状态之后，先将bHaltIsSetToTrue置为TRUE，再将各个子系统的Halt方法以TRUE调用
				IF NOT bHaltIsSetToTrue THEN
					bHaltIsSetToTrue := TRUE;
	
					fbSeparateModule.Halt(bHalt := TRUE);
					fbMetalSorting.Halt(bHalt := TRUE);
					fbPlasticSorting.Halt(bHalt := TRUE);		
				END_IF

				// 如果各个子系统未完成停止的流程，则继续以TRUE的形式继续调用各个子系统的Halt方法
				IF NOT fbSeparateModule.bState_HaltDone THEN
					fbSeparateModule.Halt(bHalt := TRUE);
				END_IF				
				IF NOT fbMetalSorting.bState_HaltDone THEN
					fbMetalSorting.Halt(bHalt := TRUE);
				END_IF			
				IF NOT fbPlasticSorting.bState_HaltDone THEN
					fbPlasticSorting.Halt(bHalt := TRUE);
				END_IF

				// 如果所有子系统都停止了，那StateComplete则为TRUE。代表中止完成。状态会经过状态机功能块自动进入ABORTED
				IF fbSeparateModule.bState_HaltDone AND fbMetalSorting.bState_HaltDone AND fbPlasticSorting.bState_HaltDone THEN
					fbStateMachineSemiAuto.StateComplete := TRUE;
				END_IF
	
	// ========================中止状态=================================
	E_PMLState.ABORTED:	

				// 进入中止状态之后，先将bHaltIsSetToTrue置回FALSE，再将各个子系统的Halt方法以FALSE调用
				IF bHaltIsSetToTrue THEN
					bHaltIsSetToTrue := FALSE;
					
					fbSeparateModule.Halt(bHalt := FALSE);
					fbMetalSorting.Halt(bHalt := FALSE);
					fbPlasticSorting.Halt(bHalt := FALSE);
				END_IF
	
				// 将StateComplete置回FALSE			
				IF fbStateMachineSemiAuto.StateComplete THEN
					fbStateMachineSemiAuto.StateComplete := FALSE;
				END_IF
	
	// =======================清除中状态================================
	E_PMLState.CLEARING:
				
				// 将StateComplete置为TRUE，这里清除中的过程是用Reseting代替
				fbStateMachineAuto.StateComplete := TRUE;
	
	// =========================正常的停止中状态================================
	E_PMLState.STOPPING:	

				// 如果检测到被分割物料的上升沿，那么nBoxesOnTheWay会加1，代表输送带上有一个物料正在运输
				IF fbTriggerSeparated.Q THEN
					nBoxesOnTheWay := nBoxesOnTheWay + 1;
				END_IF
				
				// 如果检测到金属物料被分拣完成的上升沿，那么nBoxesOnTheWay会减1，代表输送带上少了一个正在运输的物料
				IF fbTriggerSelectedM.Q THEN
					nBoxesOnTheWay := nBoxesOnTheWay - 1;
				END_IF
				
				// 如果检测到塑料物料被分拣完成的上升沿，那么nBoxesOnTheWay会减1，代表输送带上少了一个正在运输的物料
				IF fbTriggerSelectedP.Q THEN
					nBoxesOnTheWay := nBoxesOnTheWay - 1;
				END_IF
				
				// 只有当nBoxesOnTheWay为0且bHaltIsSetToTrue为FALSE（没用以TRUE调用过Halt方法）的时候，将bHaltIsSetToTrue置为TRUE
				IF (nBoxesOnTheWay = 0) AND NOT bHaltIsSetToTrue THEN
					bHaltIsSetToTrue := TRUE;				
				END_IF
				
				// 如果输送系统没用完成停止，或者输送带上仍然有物料，那么继续调用输送系统的自动方法等待该流程执行完毕。当nBoxesOnTheWay为0，以TRUE调用输送系统的Halt方法
				IF NOT fbSeparateModule.bState_HaltDone OR (nBoxesOnTheWay <> 0) THEN
					fbSeparateModule.Semiautomatic();
					
					IF (nBoxesOnTheWay = 0) THEN
						fbSeparateModule.Halt(bHalt := TRUE);
					END_IF
				END_IF

				// 如果输送系统没用完成停止，或者输送带上仍然有物料，那么继续调用输送系统的自动方法等待该流程执行完毕。当nBoxesOnTheWay为0，以TRUE调用金属分拣系统的Halt方法				
				IF NOT fbMetalSorting.bState_HaltDone OR (nBoxesOnTheWay <> 0) THEN
					fbMetalSorting.Semiautomatic();
					
					IF (nBoxesOnTheWay = 0) THEN
						fbMetalSorting.Halt(bHalt := TRUE);
					END_IF
				END_IF

				// 如果输送系统没用完成停止，或者输送带上仍然有物料，那么继续调用输送系统的自动方法等待该流程执行完毕。当nBoxesOnTheWay为0，以TRUE调用塑料分拣系统的Halt方法				
				IF NOT fbPlasticSorting.bState_HaltDone OR (nBoxesOnTheWay <> 0) THEN
					fbPlasticSorting.Semiautomatic();
					
					IF (nBoxesOnTheWay = 0) THEN
						fbPlasticSorting.Halt(bHalt := TRUE);
					END_IF
				END_IF

				// 如果各个子系统都完成停止了，且输送带上没有物料了，StateComplete才会被置为TRUE，代表停止完成。状态会经过状态机功能块自动进入STOPPED
				IF fbSeparateModule.bState_HaltDone AND fbMetalSorting.bState_HaltDone
				AND fbPlasticSorting.bState_HaltDone AND (nBoxesOnTheWay = 0) THEN
					fbStateMachineSemiAuto.StateComplete := TRUE;
				END_IF
					
	// ===========================停止状态==============================
	E_PMLState.STOPPED:	
				
				// 进入停止状态之后，先将bHaltIsSetToTrue置回FALSE，再将各个子系统的Halt方法以FALSE调用
				IF bHaltIsSetToTrue THEN
					bHaltIsSetToTrue := FALSE;
					
					fbSeparateModule.Halt(bHalt := FALSE);
					fbMetalSorting.Halt(bHalt := FALSE);
					fbPlasticSorting.Halt(bHalt := FALSE);
				END_IF
				
				// 将StateComplete置回FALSE
				IF fbStateMachineSemiAuto.StateComplete THEN
					fbStateMachineSemiAuto.StateComplete := FALSE;
				END_IF

	// =========================复位中状态================================
	E_PMLState.RESETTING:	

				// 进入复位中状态之后，先将bResetIsSetToTrue置为TRUE，再将各个子系统的Reset方法以TRUE调用
				IF NOT bResetIsSetToTrue THEN
					bResetIsSetToTrue := TRUE;
					
					fbSeparateModule.Reset(bReset := TRUE);							
					fbMetalSorting.Reset(bReset := TRUE);
					fbPlasticSorting.Reset(bReset := TRUE);
				END_IF
	
				// 如果各个子系统未完成复位的流程，则继续以TRUE的形式继续调用各个子系统的Reset方法			
				IF NOT fbSeparateModule.bState_ResetDone THEN
					fbSeparateModule.Reset(bReset := TRUE);
				END_IF				
				IF NOT fbMetalSorting.bState_ResetDone THEN
					fbMetalSorting.Reset(bReset := TRUE);
				END_IF			
				IF NOT fbPlasticSorting.bState_ResetDone THEN
					fbPlasticSorting.Reset(bReset := TRUE);
				END_IF
				
				// 如果各个子系统都完成复位了，且所有气缸都回到基始位了，那么nBoxesOnTheWay也一并清零。同时，将StateComplete置为TRUE
				IF fbSeparateModule.bState_ResetDone AND fbMetalSorting.bState_ResetDone AND fbPlasticSorting.bState_ResetDone 
				AND fbSeparateModule.bState_ClampAtBasePos AND fbSeparateModule.bState_BarrierAtBasePos
				AND fbMetalSorting.bState_CylinderAtBasePos AND fbPlasticSorting.bState_CylinderAtBasePos THEN
					nBoxesOnTheWay 							:= 0;
					fbStateMachineSemiAuto.StateComplete 	:= TRUE;
				END_IF
END_CASE

// =========================================================
END_METHOD

END_FUNCTION_BLOCK
